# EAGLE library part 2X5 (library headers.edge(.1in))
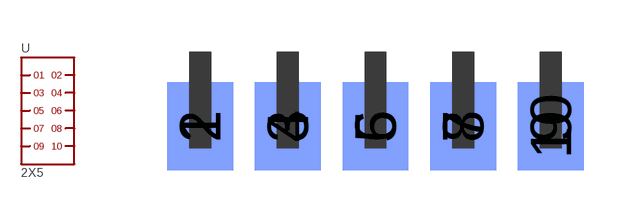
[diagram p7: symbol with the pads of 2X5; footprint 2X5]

Designator prefix -

## 2X5  [2X5]
1  1
2  2
3  3
4  4
5  5
6  6
7  7
8  8
9  9
10  10

## Footprint 2X5 (pad centres in mm)
smd 1.905 x 2.54: 1 0,-2.159; 3 2.54,-2.159; 5 5.08,-2.159; 7 7.62,-2.159; 9 10.16,-2.159
smd 1.905 x 2.54 bottom: 2 0,-2.159; 4 2.54,-2.159; 6 5.08,-2.159; 8 7.62,-2.159; 10 10.16,-2.159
